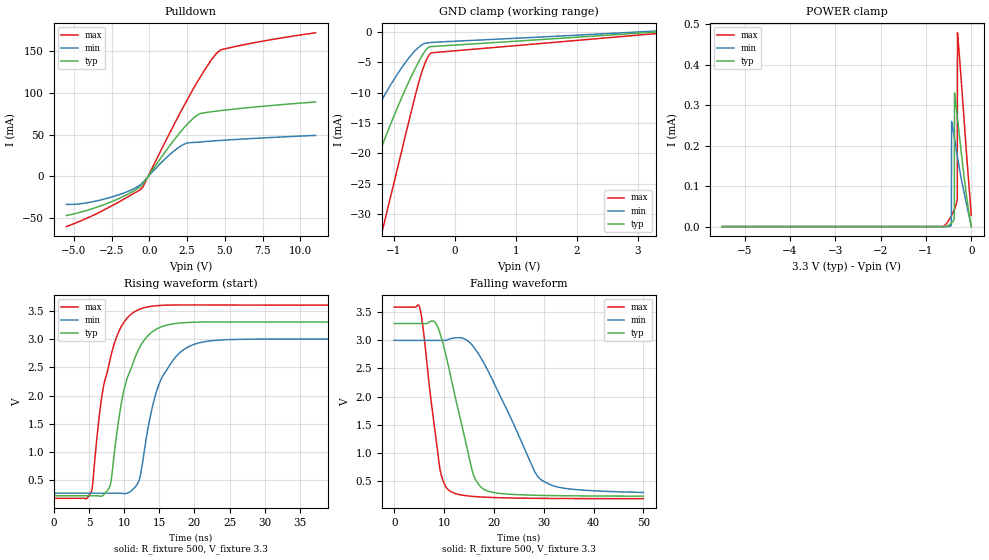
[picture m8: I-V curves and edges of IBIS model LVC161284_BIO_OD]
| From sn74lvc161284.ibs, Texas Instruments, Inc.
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[Model]   LVC161284_BIO_OD
Model_type  I/O_open_drain
Vinl=0.8
Vinh=2.0
Enable   Active-Low
Vref =   3.3
Rref =   500
Cref =   50p
Vmeas =   1.5
| variable   typ   min   max
C_comp   4.99pF   4.39pF   5.65pF
| C_pulldown   4.43pF   3.88pF   5.14pF
| C_tri-state   4.99pF   4.39pF   5.65pF
[Temperature Range]   40   100   -40
| Ambient temperature   25   85   -40
[Voltage range]   3.3   3   3.6
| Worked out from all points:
|   slope of the pulldown table from 0 to 0.495 V, typ, clamps not added: 37.8 ohm
|   rising waveform, R_fixture 500, V_fixture 3.3: 20-80 % time 3.13ns typ, 3.44ns min, 2.77ns max; typ from 0.225 V to 3.3 V
|   falling waveform, R_fixture 500, V_fixture 3.3: 20-80 % time 4.71ns typ, 8.51ns min, 2.74ns max; typ from 3.3 V to 0.227 V
[GND Clamp]
| LVC161284_BIO_OD
|   Voltage   I(typ)   I(min)   I(max)
-5.5V     -150.9mA   -105.1mA   -231.1mA
-2.265V   -49.03mA   -32.34mA   -79.17mA
-1.755V   -34.12mA   -21.78mA   -56.65mA
-1.685V   -32.13mA   -20.38mA   -53.62mA
-1.205V   -19.04mA   -11.32mA   -33.36mA
-1.15V    -17.62mA   -10.35mA   -31.1mA
-825mV    -9.746mA   -5.218mA   -17.63mA
-585mV    -4.755mA   -2.446mA   -8.044mA
-480mV    -3.025mA   -1.842mA   -4.908mA
-435mV    -2.549mA   -1.781mA   -3.991mA
-395mV    -2.411mA   -1.738mA   -3.5mA
3.3V      150.7pA    168.7uA    -261.4uA
[POWER Clamp]
| LVC161284_BIO_OD
|   Voltage   I(typ)   I(min)   I(max)
-5.5V     46.92nA    131.6nA    6.247nA
-585mV    12.2nA     2.725nA    3.285uA
-440mV    8.724uA    2.432uA    26.26uA
-435mV    9.268uA    259.4uA    27.35uA
-375mV    19.07uA    220.6uA    42.01uA
-370mV    330uA      217.2uA    43.39uA
-310mV    273uA      175.6uA    67.35uA
-305mV    267.9uA    172.1uA    478.3uA
-250mV    212.1uA    135.7uA    403.5uA
-130mV    96.77uA    68.64uA    218.4uA
-70mV     47.77uA    37uA       127.7uA
-95.1fV   150.7pA    776.1pA    27.84uA
[Pulldown]
| LVC161284_BIO_OD
|   Voltage   I(typ)   I(min)   I(max)
-5.5V     -46.7mA    -33.42mA   -59.97mA
-2.72V    -31.74mA   -25.77mA   -37.32mA
-1.275V   -19.72mA   -16.73mA   -22.76mA
-480mV    -10.32mA   -8.029mA   -13.64mA
1.565V    41.96mA    29.5mA     59.61mA
2.25V     57.29mA    38.13mA    83.15mA
2.75V     66.96mA    40.53mA    99.64mA
3.395V    75.38mA    41.18mA    119.7mA
4.12V     77.46mA    42.37mA    139.8mA
4.62V     78.59mA    43mA       150.1mA
6.93V     83.02mA    45.54mA    160mA
11V       89.16mA    49.12mA    171.9mA
[Ramp]
| LVC161284_BIO_OD
| variable   typ   min   max
dV/dt_r   1.85/3.13E-09   1.64/3.44E-09   2.06/2.77E-09
dV/dt_f   1.87/4.79E-09   1.65/8.68E-09   2.07/2.77E-09
R_load = 500
[Rising Waveform]
| LVC161284_BIO_OD
R_fixture =   500
C_fixture =   0
L_fixture =   0
V_fixture =   3.3
V_fixture_min = 3
V_fixture_max = 3.6
|   Time   V(typ)   V(min)   V(max)
0s        225.3mV    271.6mV    181mV
5.32ns    225.3mV    271.6mV    293.3mV
6.73ns    217.8mV    271.6mV    1.901V
7.825ns   354.9mV    271.6mV    2.539V
9.82ns    2.005V     266.6mV    3.269V
11.67ns   2.707V     395.5mV    3.497V
12.28ns   2.867V     566.3mV    3.532V
14.91ns   3.196V     2.184V     3.593V
19ns      3.294V     2.855V     3.605V
50ns      3.301V     3V         3.6V
[Falling Waveform]
| LVC161284_BIO_OD
R_fixture =   500
C_fixture =   0
L_fixture =   0
V_fixture =   3.3
V_fixture_min = 3
V_fixture_max = 3.6
|   Time   V(typ)   V(min)   V(max)
0s        3.3V       3V         3.592V
5.105ns   3.3V       3V         3.586V
5.81ns    3.3V       3V         3.207V
7.91ns    3.343V     3V         1.577V
9.145ns   3.138V     3V         730mV
11.04ns   2.48V      3.021V     327.3mV
15.75ns   648mV      2.904V     222.8mV
17.88ns   354.9mV    2.615V     210.2mV
29.32ns   240.7mV    529.2mV    187.3mV
50ns      226.9mV    293.3mV    181.6mV
